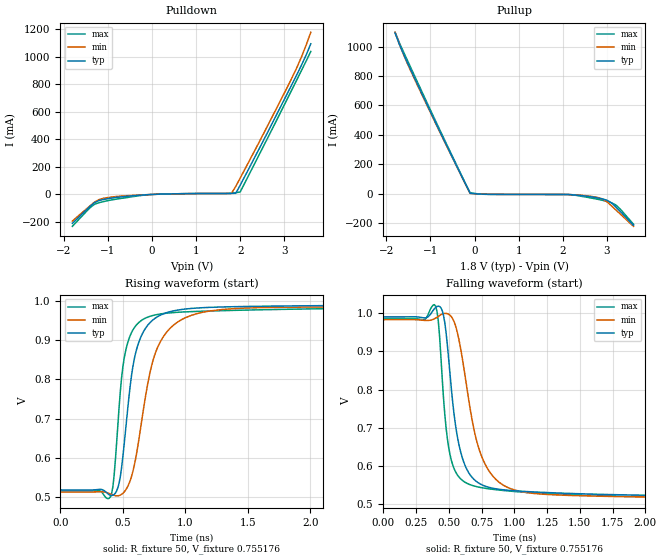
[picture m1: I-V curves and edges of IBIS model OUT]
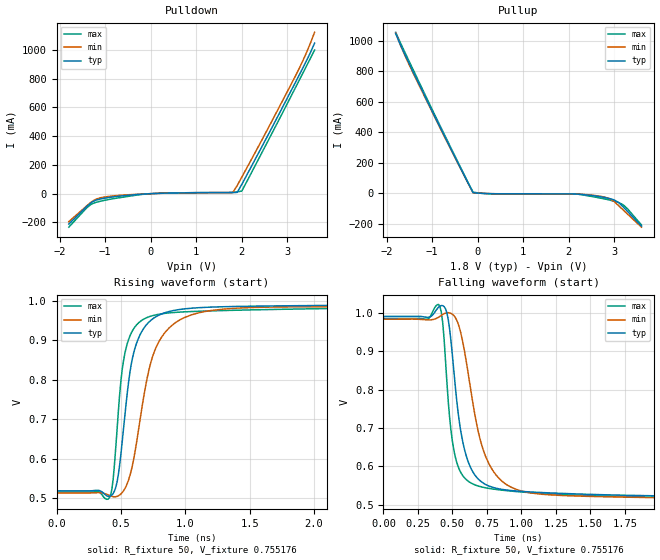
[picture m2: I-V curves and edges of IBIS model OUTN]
|   IBIS File of SG2520VHN E
|   LVDS, Vcc=1.8V, Io=4.5mA, fo>212.5MHz
[IBIS Ver]   3.2
[File Name]   sg2520vhn_hf_45m_18v.ibs
[File Rev]   1.0
[Date]   July 29, 2020
[Source]
Fairchild Ensigna Lab's Method
[Notes]
Created by Minoru Kozaki
[Disclaimer]
Seiko Epson Corporation makes no warranty with respect to the
information contained herein.
[Copyright]
Copyright(C) 2020, Seiko Epson Corporation. All rights reserved.
|   Component
[Component]   SG2520VHN
[Manufacturer]  Seiko Epson Corporation
[Package]
R_pkg   17.7m   NA   NA
L_pkg   235p   NA   NA
C_pkg   208f   NA   NA
[Pin]   signal_name   model_name   R_pin   L_pin   C_pin
1   OE/ST   NC
2   NC   NC
3   GND   GND
4   OUT   OUT   17.7m   235p   208f
5   OUTN   OUTN   10.4m   129p   221f
6   VCC   POWER
[Diff Pin] inv_pin  vdiff  tdelay_typ
4   5   0   0
| Models and submodels in the file (2): OUT (Output), OUTN (Output)
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|   Model OUT
[Model]   OUT
Model_type   Output
Polarity   Non-Inverting
Vref = 0.75
Vmeas = 0.75
Rref = 50
Cref = 0
C_comp   4.5p   4.5p   4.5p
[Temperature Range]   25   105   -40
[Voltage Range]   1.8   1.71   1.89
[Pullup Reference]   1.8   1.71   1.89
[Pulldown Reference]   0   0   0
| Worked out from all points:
|   slope of the pulldown table from 0 to 0.27 V, typ, clamps not added: 83.5 ohm
|   slope of the pullup table from 0 to 0.27 V, typ, clamps not added: 64.4 ohm
|   falling waveform, R_fixture 50, V_fixture 0.755176: 20-80 % time 116ps typ, 173ps min, 84.8ps max; typ from 0.99 V to 0.52 V
|   rising waveform, R_fixture 50, V_fixture 0.755176: 20-80 % time 126ps typ, 182ps min, 93.2ps max; typ from 0.519 V to 0.99 V
[Pullup]
-1.8V     1.091A     1.097A     1.096A
-1.6V     943.2mA    939.1mA    957.4mA
-1.4V     812.9mA    804.9mA    827.3mA
-800mV    431.9mA    427mA      441.7mA
-100mV    2.885mA    1.852mA    6.305mA
300mV     -4.211mA   -3.624mA   -4.287mA
2.1V      -5.427mA   -5.538mA   -5.243mA
2.8V      -29.27mA   -26.73mA   -38.5mA
3V        -44.42mA   -55.23mA   -52.86mA
3.1V      -61.72mA   -82.26mA   -61.57mA
3.2V      -90.17mA   -110.2mA   -76.52mA
3.6V      -214.6mA   -221.4mA   -207.4mA
[Pulldown]
-1.8V     -209.8mA   -192.9mA   -230.9mA
-1.4V     -86.58mA   -82.28mA   -95.93mA
-1.3V     -59.74mA   -55.67mA   -71.78mA
-1.2V     -44.44mA   -37.58mA   -59.85mA
-1V       -30.66mA   -22.68mA   -45.13mA
0V        -69.43uA   -62.02uA   -71.92uA
1.8V      7.275mA    6.88mA     9.342mA
1.9V      8.59mA     58.38mA    12.84mA
2V        66.5mA     118.5mA    17.82mA
3.2V      816.1mA    863.5mA    778mA
3.4V      945.4mA    1.006A     906.5mA
3.6V      1.093A     1.176A     1.037A
[Falling Waveform]
R_fixture = 50
V_fixture = 0.755176
V_fixture_min = 0.748585
V_fixture_max = 0.751033
0s        990.3mV    983.1mV    985mV
390ps     1.012V     985.3mV    1.022V
440ps     1.014V     996.1mV    887.5mV
470ps     975.3mV    999.6mV    734.9mV
510ps     839.8mV    994.5mV    629.5mV
580ps     652.5mV    927.1mV    570.4mV
670ps     573.7mV    736.5mV    550.3mV
800ps     544.8mV    590.9mV    540.6mV
1.05ns    534.1mV    533.2mV    532mV
4ns       519.6mV    514.5mV    516.4mV
[Rising Waveform]
R_fixture = 50
V_fixture = 0.755176
V_fixture_min = 0.748585
V_fixture_max = 0.751033
0s        519.2mV    513.7mV    516.1mV
390ps     506.9mV    510.3mV    497.7mV
450ps     516.7mV    504.1mV    639.6mV
490ps     576.8mV    508.2mV    805.7mV
530ps     698mV      522.9mV    883.3mV
600ps     864.4mV    595.2mV    935.1mV
700ps     938.1mV    790.7mV    958.3mV
840ps     968.4mV    915.8mV    967.9mV
1.15ns    982.4mV    971.3mV    973.4mV
4ns       989.9mV    983.2mV    984.2mV
[Ramp]
R_load = 50
dV/dt_r   0.28264/126.50p   0.28058/181.11p   0.28184/94.02p
dV/dt_f   0.28264/115.75p   0.28058/172.28p   0.28184/84.65p
|   Model OUTN
[Model]   OUTN
Model_type   Output
Polarity   Inverting
Vref = 0.75
Vmeas = 0.75
Rref = 50
Cref = 0
C_comp   4.5p   4.5p   4.5p
[Temperature Range]   25   105   -40
[Voltage Range]   1.8   1.71   1.89
[Pullup Reference]   1.8   1.71   1.89
[Pulldown Reference]   0   0   0
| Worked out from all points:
|   slope of the pulldown table from 0 to 0.27 V, typ, clamps not added: 83.4 ohm
|   slope of the pullup table from 0 to 0.27 V, typ, clamps not added: 64.4 ohm
|   falling waveform, R_fixture 50, V_fixture 0.755176: 20-80 % time 115ps typ, 171ps min, 84.9ps max; typ from 0.99 V to 0.52 V
|   rising waveform, R_fixture 50, V_fixture 0.755176: 20-80 % time 126ps typ, 181ps min, 93.5ps max; typ from 0.519 V to 0.99 V
[Pullup]
-1.8V     1.046A     1.049A     1.054A
-1.6V     909.4mA    903.9mA    923.8mA
-1.4V     784.6mA    776.7mA    798.5mA
-800mV    416.7mA    412.1mA    426.2mA
-100mV    2.89mA     1.854mA    6.309mA
300mV     -4.213mA   -3.626mA   -4.287mA
2.1V      -5.427mA   -5.541mA   -5.243mA
2.8V      -29.6mA    -26.97mA   -38.88mA
3V        -44.83mA   -55.59mA   -53.45mA
3.1V      -62.13mA   -82.89mA   -62.22mA
3.2V      -90.81mA   -111.1mA   -77.04mA
3.6V      -216.5mA   -223.3mA   -209.1mA
[Pulldown]
-1.8V     -212mA     -194.9mA   -233.3mA
-1.4V     -87.47mA   -83.17mA   -96.73mA
-1.3V     -60.24mA   -56.23mA   -72.29mA
-1.2V     -44.75mA   -37.91mA   -60.26mA
-1V       -30.85mA   -22.89mA   -45.41mA
0V        -69.47uA   -62.02uA   -71.97uA
1.8V      7.276mA    7.223mA    9.341mA
1.9V      8.587mA    56.61mA    12.82mA
2V        64.24mA    114.6mA    17.78mA
3.2V      787.7mA    832.7mA    750.9mA
3.4V      911.6mA    965.9mA    874.9mA
3.6V      1.048A     1.123A     1A
[Falling Waveform]
R_fixture = 50
V_fixture = 0.755176
V_fixture_min = 0.748585
V_fixture_max = 0.751033
0s        990.4mV    983.2mV    985mV
400ps     1.014V     988.3mV    1.021V
450ps     1.011V     999mV      877.2mV
480ps     957.9mV    999.7mV    727.6mV
520ps     813mV      988.3mV    626.5mV
580ps     656.3mV    915.3mV    573.9mV
680ps     570.2mV    703.2mV    550mV
820ps     543mV      576.3mV    540mV
1.05ns    533.9mV    532.2mV    532.1mV
4ns       519.5mV    514.4mV    516.3mV
[Rising Waveform]
R_fixture = 50
V_fixture = 0.755176
V_fixture_min = 0.748585
V_fixture_max = 0.751033
0s        519.1mV    513.6mV    516mV
400ps     505.2mV    508.9mV    498.1mV
440ps     512.4mV    504.4mV    549mV
480ps     559.7mV    506.5mV    718.3mV
530ps     706.7mV    524.2mV    865mV
600ps     868.4mV    600.5mV    929.1mV
720ps     946.2mV    827.5mV    959.2mV
880ps     972.6mV    932.4mV    968.9mV
1.2ns     983.4mV    974.8mV    973.9mV
4ns       990mV      983.4mV    984.3mV
[Ramp]
R_load = 50
dV/dt_r   0.28235/125.81p   0.28032/179.07p   0.28155/94.29p
dV/dt_f   0.28235/114.69p   0.28032/169.78p   0.28155/84.50p
